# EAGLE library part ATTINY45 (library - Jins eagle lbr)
Atmel 8-pin 2/4/8kB flash uC
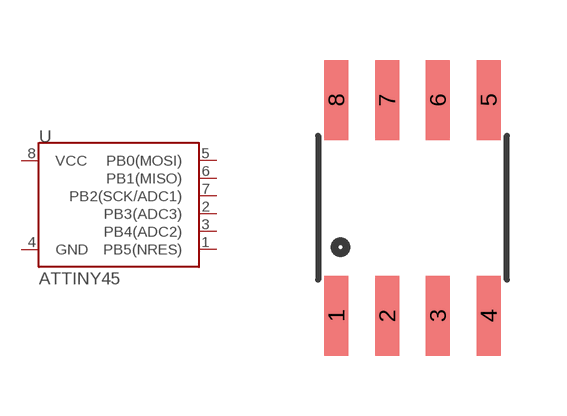
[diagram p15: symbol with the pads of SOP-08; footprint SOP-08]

Designator prefix U

## ATTINY45-TINY85  [SOP-08]
1  PB5(NRES)
2  PB3(ADC3)
3  PB4(ADC2)
4  GND
5  PB0(MOSI)
6  PB1(MISO)
7  PB2(SCK/ADC1)
8  VCC

## Footprint SOP-08 (pad centres in mm)
smd 0.6 x 2: 1 -1.905,-2.7; 2 -0.635,-2.7; 3 0.635,-2.7; 4 1.905,-2.7; 5 1.905,2.7; 6 0.635,2.7; 7 -0.635,2.7; 8 -1.905,2.7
